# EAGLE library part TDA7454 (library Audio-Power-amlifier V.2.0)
The TDA7454 is a new BCD technology QUAD BRIDGE type of car radio amplifier in Flexiwatt25 packagespecially intendedfor car radio applications. Among the features, its superior efficiency performance coming from the internal exclusive structure, makes it the most suitable device to simplify the thermal management in high power sets. The dissipated output power under average listening condition is in fact reduced up to 50% when compared to the level provided by conventional class AB solutions.
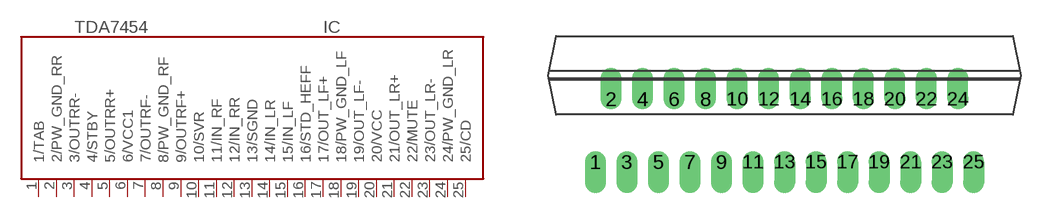
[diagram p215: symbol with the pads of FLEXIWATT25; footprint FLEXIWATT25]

Designator prefix IC

## TDA7454  [FLEXIWATT25]
1  1/TAB  in
2  2/PW_GND_RR  pwr
3  3/OUTRR-  out
4  4/STBY  in
5  5/OUTRR+  out
6  6/VCC1  pwr
7  7/OUTRF-  out
8  8/PW_GND_RF  pwr
9  9/OUTRF+  out
10  10/SVR  in
11  11/IN_RF  in
12  12/IN_RR  in
13  13/SGND  pwr
14  14/IN_LR  in
15  15/IN_LF  in
16  16/STD_HEFF
17  17/OUT_LF+  out
18  18/PW_GND_LF  pwr
19  19/OUT_LF-  out
20  20/VCC  pwr
21  21/OUT_LR+  out
22  22/MUTE  in
23  23/OUT_LR-  out
24  24/PW_GND_LR  pwr
25  25/CD

## Footprint FLEXIWATT25 (pad centres in mm)
Flexiwatt25 (vertical)
drill 0.813 offset: 1 -12,0; 2 -11,4; 3 -10,0; 4 -9,4; 5 -8,0; 6 -7,4; 7 -6,0; 8 -5,4; 9 -4,0; 10 -3,4; 11 -2,0; 12 -1,4; 13 0,0; 14 1,4; 15 2,0; 16 3,4; 17 4,0; 18 5,4; 19 6,0; 20 7,4; 21 8,0; 22 9,4; 23 10,0; 24 11,4; 25 12,0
